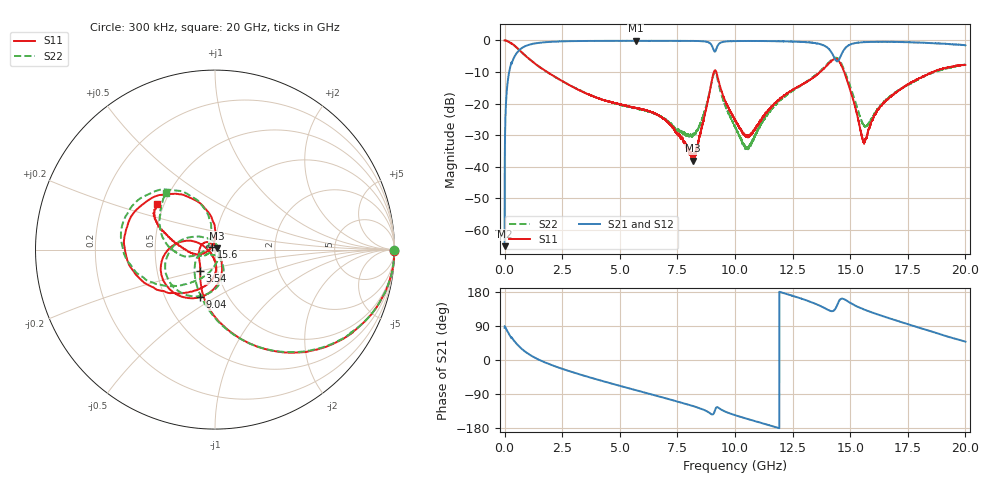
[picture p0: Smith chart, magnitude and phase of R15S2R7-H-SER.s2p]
!{R15S2R7}
!Johanson Technology Inc.
!www.johansontechnology.com
!Test Board Conditions:
!Substrate Type  RO4350B
!Substrate Thickness  20 mil
!Substrate Dk  3.66
!TL Type: GCPW
!TL Trace Width  34 mil
!TL Gap  10 mil
!Electrode orientation  Horizontal
!DUT TOPOLOGY	SERIES
!Mounting Pad LxW  26x52 mil
! Created Sat Feb  6 13:52:09 2021
# hz S ma R 50
! 2 Port Network Data from SP1.SP block
! freq  magS11  angS11  magS21  angS21  magS12  angS12  magS22  angS22
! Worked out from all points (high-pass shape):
!   20001 points, 300 kHz to 20 GHz, reference 50 ohm
!   highest |S21| = -0.11 dB at 5.692 GHz (marker M1); lowest = -65.2 dB at 300 kHz (marker M2)
!   |S21| within 3 dB of the highest: 629.5 MHz to 9.079 GHz (8.45 GHz wide, 174 % of centre); 14.72 GHz to end of sweep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
!   lowest |S11| = -38.1 dB at 8.156 GHz (marker M3), VSWR 1.03, Z = 51.1 + j0.669 ohm
!   |S11| at or under -10 dB: 1.848 GHz to 9.083 GHz (7.235 GHz wide, 132 % of centre); 9.188 GHz to 13.7 GHz (4.509 GHz wide, 39.4 % of centre); 14.74 GHz to 18.61 GHz (3.869 GHz wide, 23.2 % of centre)
!   |S22| runs from -34.6 to 0.0 dB; largest |S21 - S12| = 0.013
!   S11 on the Smith chart (normalised r, x): 300 kHz: open; 3.54 GHz: 0.82, -0.20; 9.04 GHz: 0.74, -0.43; 15.6 GHz: 0.96, +0.03; 20 GHz: 0.46, +0.28
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300000  1 -0.3  0.00055 85.3  0.0004838 91.5  0.9968 -0.2
1.273e8  0.9765 -14.3  0.211 75.4  0.2118 75.4  0.9756 -14.2
4.463e8  0.8188 -41.7  0.5697 48.1  0.5713 48.2  0.8175 -41.4
1.4243e9  0.4028 -86.6  0.9096 2.7  0.9095 2.6  0.4011 -87.4
3.3343e9  0.1572 -121.6  0.9807 -39.3  0.9797 -39.4  0.158 -136.2
3.5403e9  0.1453 -124.7  0.981 -43.0  0.9812 -43.1  0.1457 -140.6
5.6923e9  0.08516 176.5  0.9875 -79.6  0.9855 -79.6  0.08388 -154.7
6.6673e9  0.06563 140.8  0.9855 -95.6  0.9857 -95.6  0.06595 -149.8
8.1563e9  0.01248 31.6  0.9827 -121.1  0.9827 -121.1  0.03102 -92.1
8.5813e9  0.04561 -50.2  0.9742 -129.9  0.9741 -129.8  0.05947 -61.1
9.0403e9  0.2784 -107.7  0.7598 -143.5  0.7613 -143.5  0.2635 -104.6
9.3503e9  0.188 166.0  0.912 -128.8  0.9129 -129.0  0.1672 157.0
1.00003e10  0.05452 167.4  0.9774 -145.5  0.9772 -145.5  0.04281 96.1
1.05473e10  0.03123 -141.5  0.9802 -155.6  0.9816 -155.6  0.01937 11.7
1.16723e10  0.09569 -86.4  0.9744 -175.5  0.974 -175.5  0.08822 -90.5
1.33343e10  0.2495 -114.9  0.9227 152.2  0.9258 152.1  0.2541 -130.6
1.40453e10  0.4209 -151.9  0.7491 132.0  0.7573 131.7  0.4346 -160.0
1.44993e10  0.4737 147.9  0.4864 153.8  0.488 153.8  0.5035 145.3
1.49063e10  0.2095 99.9  0.8257 154.5  0.8227 154.5  0.2345 104.5
1.56033e10  0.02302 144.0  0.9398 133.1  0.9361 133.3  0.04535 140.2
1.66673e10  0.1208 -169.4  0.9532 110.6  0.9447 110.7  0.1242 -164.1
2e10  0.4103 141.5  0.8382 48.4  0.8299 48.1  0.4158 130.4
